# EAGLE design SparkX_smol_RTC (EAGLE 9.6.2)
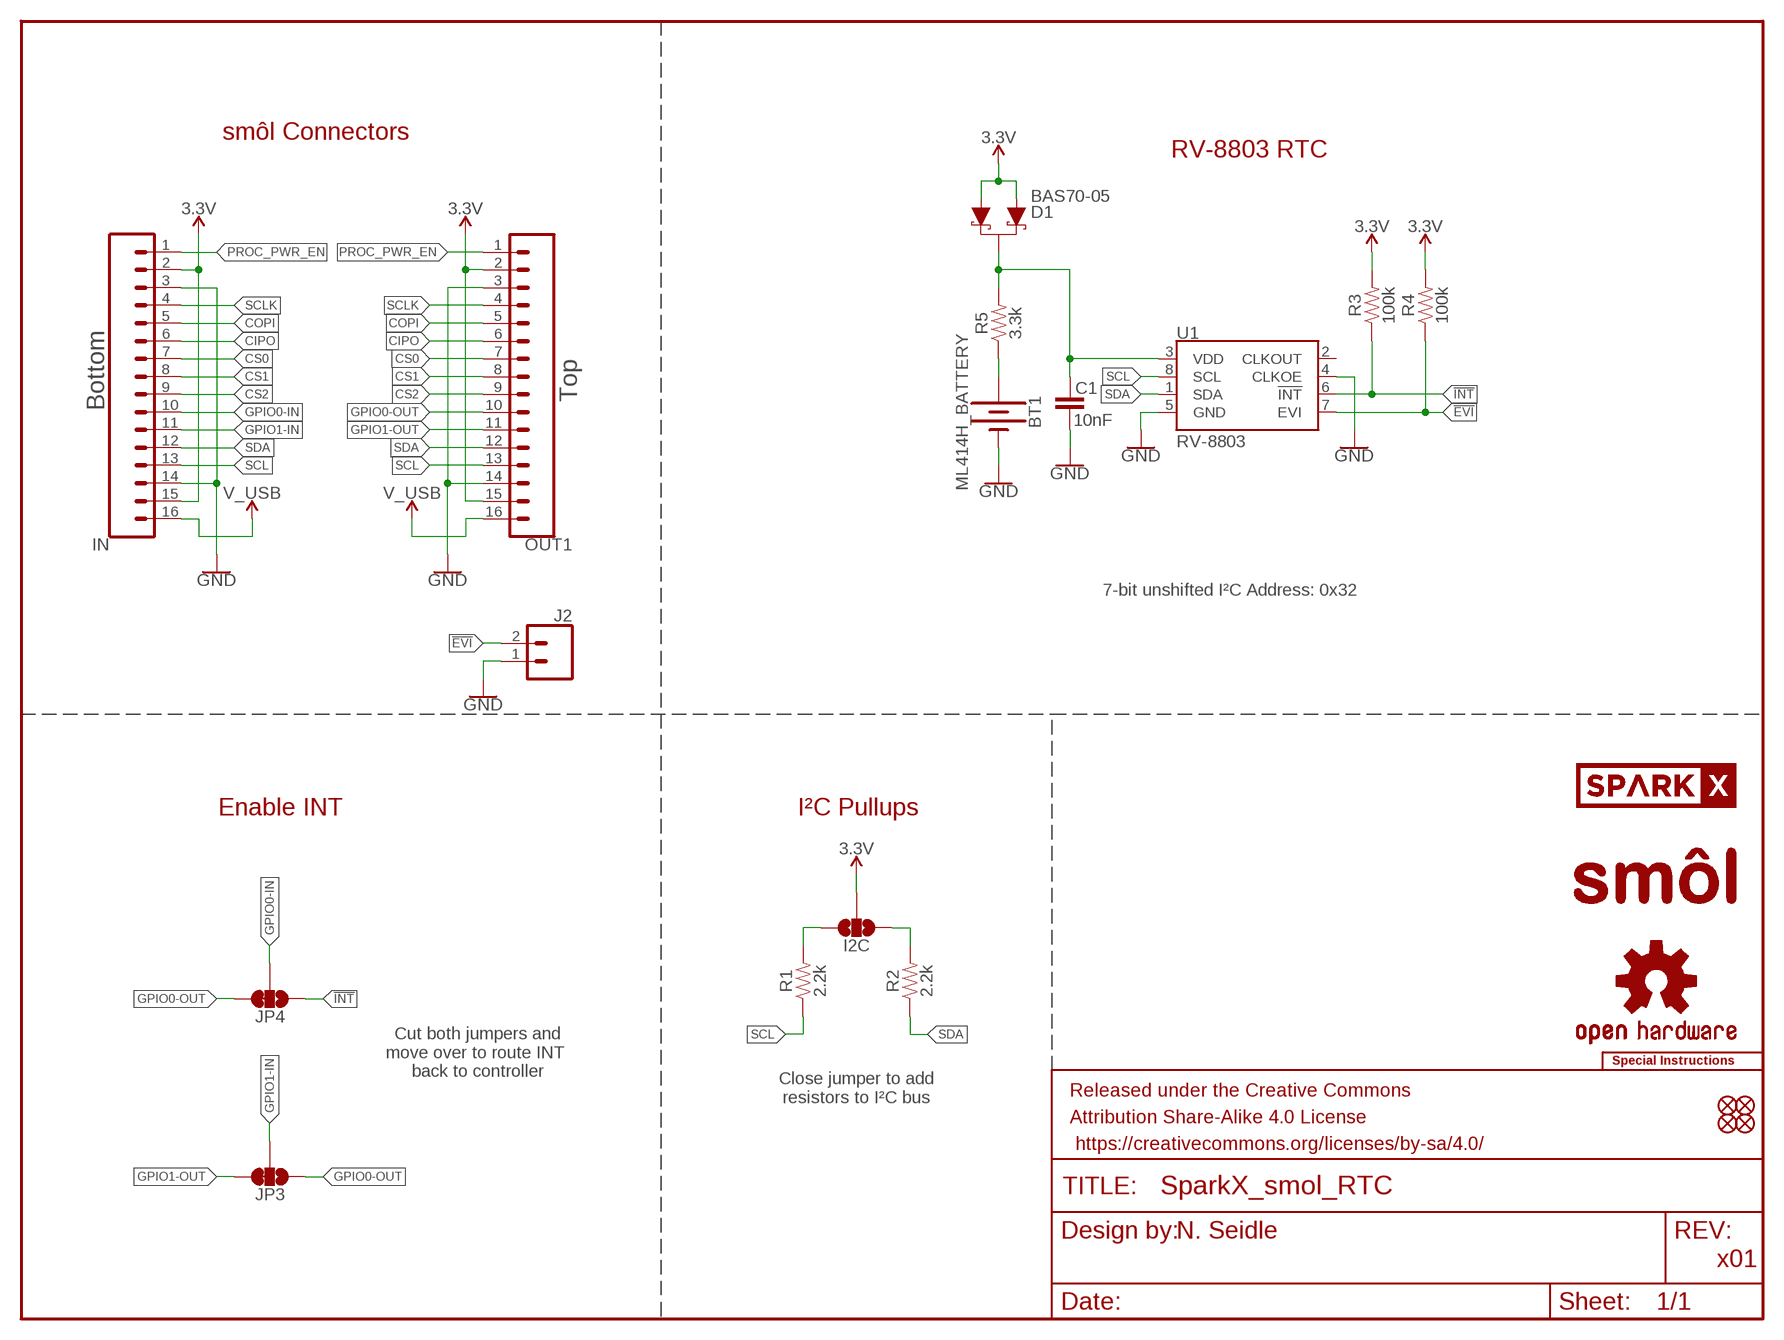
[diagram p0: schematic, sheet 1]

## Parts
BT1  ML414H_BATTERY  ML414H_IV01E_BATTERY  [ML414H_IV01E]
C1  10nF  10NF-0603-50V-10%  [0603]
D1  BAS70-05  DIODE-SCHOTTKY-DUAL  [SOT23-3@1]
FD1  FIDUCIALUFIDUCIAL  [FIDUCIAL-MICRO]
FD2  FIDUCIALUFIDUCIAL  [FIDUCIAL-MICRO]
FD3  FIDUCIALUFIDUCIAL  [FIDUCIAL-MICRO]
FD4  FIDUCIALUFIDUCIAL  [FIDUCIAL-MICRO]
FRAME2  FRAME-LETTER  [CREATIVE_COMMONS]
I2C  JUMPER-SMT_3_NO_SILK  [SMT-JUMPER_3_NO_SILK]
IN  CONN_16FPC_16_0.5MM  [FPC_16_0.5MM]
J2  CONN_021X02_NO_SILK  [1X02_NO_SILK]
JP3  JUMPER-SMT_3_1-NC_TRACE_SILK  [SMT-JUMPER_3_1-NC_TRACE_SILK]
JP4  JUMPER-SMT_3_1-NC_TRACE_SILK  [SMT-JUMPER_3_1-NC_TRACE_SILK]
LOGO1  SPECIAL_INSTRUCTIONS-ORDERING  [ORDERING_INSTRUCTIONS]
LOGO2  OSHW-LOGOMINI  [OSHW-LOGO-MINI]
OUT1  CONN_16FPC_16_0.5MM  [FPC_16_0.5MM]
R1  2.2k  2.2KOHM-0603-1/10W-1%  [0603@1]
R2  2.2k  2.2KOHM-0603-1/10W-1%  [0603@1]
R3  100k  100KOHM-0603-1/10W-1%  [0603@2]
R4  100k  100KOHM-0603-1/10W-1%  [0603@2]
R5  3.3k  3.3KOHM-0603-1/10W-1%  [0603]
U1  RV-8803  [RV-3028]
U$1  SPARKX-LOGO3  [SPARKX-SMALL]
U$39  SMOL_LOGOSMALL  [SMOL_SMALL]

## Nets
3.3V [power]: D1.1(A) D1.2(A1) I2C.2 IN.2 IN.15 OUT1.2 OUT1.15 R3.2 R4.2
!EVI: J2.2 R4.1 U1.7(EVI)
!INT: JP4.1 R3.1 U1.6(!INT)
CIPO: IN.6 OUT1.6
COPI: IN.5 OUT1.5
CS0: IN.7 OUT1.7
CS1: IN.8 OUT1.8
CS2: IN.9 OUT1.9
GND [power]: BT1.- C1.1 IN.3 IN.14 J2.1 OUT1.3 OUT1.14 U1.4(CLKOE) U1.5(GND)
GPIO0-IN: IN.10 JP4.2
GPIO0-OUT: JP3.1 JP4.3 OUT1.10
GPIO1-IN: IN.11 JP3.2
GPIO1-OUT: JP3.3 OUT1.11
N$1: I2C.3 R1.2
N$2: I2C.1 R2.2
N$4: BT1.+ R5.1
PROC_PWR_EN: IN.1 OUT1.1
SCL: IN.13 OUT1.13 R1.1 U1.8(SCL)
SCLK: IN.4 OUT1.4
SDA: IN.12 OUT1.12 R2.1 U1.1(SDA)
V_BACKUP: C1.2 D1.3(C) R5.2 U1.3(VDD)
V_USB [power]: IN.16 OUT1.16
Unconnected: U1.2(CLKOUT)

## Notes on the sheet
- smôl Connectors
- RV-8803 RTC
- Top
- Bottom
- 7-bit unshifted I²C Address: 0x32
- Enable INT | I²C Pullups
- Cut both jumpers and
  move over to route INT 
  back to controller
- Close jumper to add
  resistors to I²C bus
- N. Seidle
- x01

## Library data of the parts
BT1 = SparkFun-Batteries:ML414H_IV01E_BATTERY: SEIKO ML414H-IV01E Reflowable Lithium Battery; PROD_ID: BATT-14267
C1 = SparkFun-Capacitors:10NF: 0.01uF/10nF/10,000pF ceramic capacitors; PROD_ID: CAP-00867
D1 = SparkFun-DiscreteSemi:DIODE-SCHOTTKY-DUAL: Diodes Incorporated - BAS70-05 Dual Schottky Diode Two Schottky Diodes in a single SOT-23 package. Low reverse current (100 nA) Vf: Datasheet referenced for footprint; PROD_ID: DIO-14829
FD1-FD4 = SparkFun-Aesthetics:FIDUCIAL: Fiducial Alignment Points
FRAME2 = SparkFun-Aesthetics:FRAME-LETTER: Schematic Frame - Letter
I2C = SparkFun-Jumpers:JUMPER-SMT_3_NO: Normally open jumper This jumper has three pads in close proximity to each other. Apply solder to close the connection(s).
IN OUT1 = SparkFun-Connectors:CONN_16: Multi connection point. Often used as Generic Header-pin footprint for 0.1 inch spaced/style header connections On any of the 0.1 inch spaced packages, you can populate with these: Break Away Headers - Straight (PRT-00116) Break Away Male Headers - Right Angle (PRT-00553) Female Headers (PRT-00115)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; PROD_ID: CONN-16066
J2 = SparkFun-Connectors:CONN_02: Multi connection point. Often used as Generic Header-pin footprint for 0.1 inch spaced/style header connections
JP3 JP4 = SparkFun-Jumpers:JUMPER-SMT_3_1-NC_TRACE: Normally closed trace jumper (1 of 2 connections) This jumper has a trace between two pads so it's normally closed (NC). The other connection is normally open (NO). Use a razor knife to open the connection. For best results follow the IPC guidelines for cutting traces: Cutout at least 0.063 mm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
LOGO1 = SparkFun-Aesthetics:SPECIAL_INSTRUCTIONS: Special Ordering/Production Instructions Alert
LOGO2 = SparkFun-Aesthetics:OSHW-LOGO: Open-Source Hardware (OSHW) Logo
R1 R2 = SparkFun-Resistors:2.2KOHM: 2.2kΩ resistor; PROD_ID: RES-08272
R3 R4 = SparkFun-Resistors:100KOHM: 100kΩ resistor; PROD_ID: RES-07828
R5 = SparkFun-Resistors:3.3KOHM: 3.3kΩ resistor; PROD_ID: RES-07851
U1 = SparkFun-Clocks:RV-8803: Micro Crystal RV-8803 - Temperature compensated RTC Ultra accurate plus/minus 3PPM I2C RTC. Temperature compensated crystal for low drift; PROD_ID: IC-14828
U$1 = SparkX:SPARKX-LOGO
U$39 = SparkX:SMOL_LOGO

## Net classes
1 power: width 0.178 mm
2 3.3V: width 0.305 mm
3 VDDA: width 0.254 mm

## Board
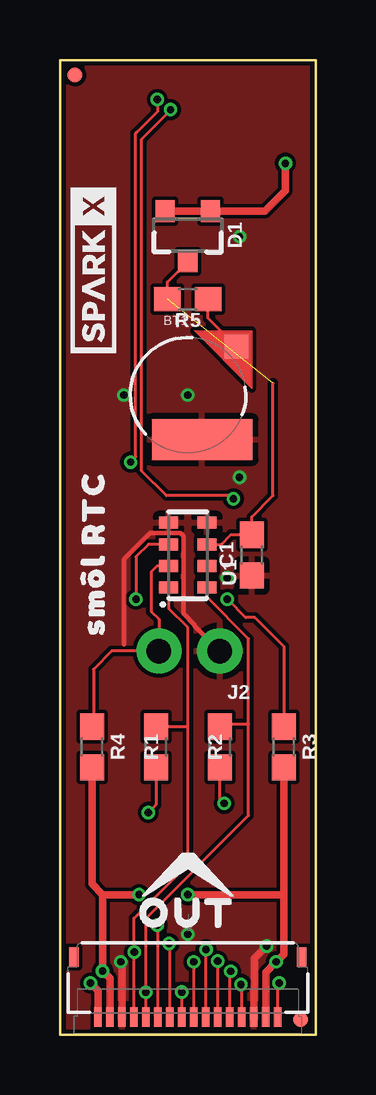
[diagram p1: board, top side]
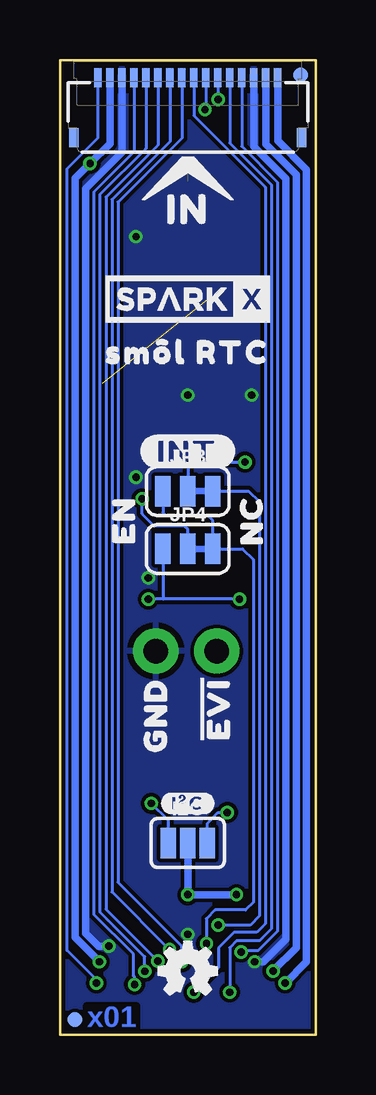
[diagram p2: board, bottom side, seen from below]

Size 10.67 x 40.64 mm. Coordinates in mm from the lower left corner, seen from the top.
Outline: 0,40.64 0,0 10.67,0 10.67,40.64 0,40.64
Copper layers (1*16): Top/Horz 0.035mm / dielectric 1.5mm / Bottom/Vert 0.035mm
Design rules "SparkFun-2-Layer-Minimum-JLCPCB": minimum track width 5mil, minimum drill 0.3mm, track to track 5mil, track to pad 5mil, pad to pad 5mil, via to via 5mil, smd to smd 5mil, copper to edge 7mil, drill to drill 7mil, minimum pad ring 5mil, minimum via ring 5mil, stop-mask expansion 2.5mil, vias tented up to drill 25mil, thermal gap 10mil

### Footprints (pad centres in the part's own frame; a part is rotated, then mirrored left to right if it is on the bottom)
ML414H_IV01E = smd 1 x 1: + 2.022,2.032 | smd 4.2 x 1.7: - 0.6,-1.85
0603 = smd 1.1 x 1: 1 -0.85,0; 2 0.85,0
SOT23-3@1 = smd 0.8 x 0.9: 1 -0.95,-1; 2 0.95,-1; 3 0,1.1
FIDUCIAL-MICRO = smd 0.635 x 0.635: 1 0,0
SMT-JUMPER_3_NO_SILK = smd 0.635 x 1.27: 1 -0.813,0; 2 0,0; 3 0.813,0
FPC_16_0.5MM = smd 0.3 x 0.8: 1 -3.75,1.35; 2 -3.25,1.35; 3 -2.75,1.35; 4 -2.25,1.35; 5 -1.75,1.35; 6 -1.25,1.35; 7 -0.75,1.35; 8 -0.25,1.35; 9 0.25,1.35; 10 0.75,1.35; 11 1.25,1.35; 12 1.75,1.35; 13 2.25,1.35; 14 2.75,1.35; 15 3.25,1.35; 16 3.75,1.35 | smd 0.4 x 0.8: MP1 -4.75,-1.15; MP2 4.75,-1.15
1X02_NO_SILK = drill 1.016 pad 1.88: 1 0,0; 2 2.54,0
SMT-JUMPER_3_1-NC_TRACE_SILK = smd 0.66 x 1.27: 1 -1.041,0; 2 0,0; 3 1.041,0
0603@1 = smd 1.1 x 1: 1 -0.85,0; 2 0.85,0
0603@2 = smd 1.1 x 1: 1 -0.85,0; 2 0.85,0
RV-3028 = smd 0.5 x 0.8: 1 -1.35,-0.8; 2 -0.45,-0.8; 3 0.45,-0.8; 4 1.35,-0.8; 5 1.35,0.8; 6 0.45,0.8; 7 -0.45,0.8; 8 -1.35,0.8

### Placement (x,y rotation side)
BT1  5.33,26.67 0 top
C1  8,20 90 top
D1  5.33,33.34 180 top
FD1  0.64,40.01 0 top
FD2  0.64,40.01 0 bottom
FD3  10.03,0.64 0 top
FD4  10.03,0.64 0 bottom
FRAME2  not placed on the board
I2C  5.33,8 0 bottom
IN  5.33,38.54 0 bottom
J2  6.67,16 180 top
JP3  5.33,22.67 0 bottom
JP4  5.33,20.26 0 bottom
LOGO1  not placed on the board
LOGO2  5.33,2.67 0 bottom
OUT1  5.33,2.1 180 top
R1  4,12 270 top
R2  6.67,12 270 top
R3  9.33,12 270 top
R4  1.33,12 270 top
R5  5.33,30.67 180 top
U1  5.33,20 90 top
U$1  1.4,31.88 90 top
U$2  [#EVI#0]  4.19,13.59 90 bottom
U$3  [GND0]  6.67,13.34 90 bottom
U$4  [SM�L_RTC0]  1.4,20.08 90 top
U$5  [SM�L_RTC0]  5.35,28.45 0 bottom
U$12  [IN0]  5.33,34.42 0 bottom
U$14  [EN1]  8,21.46 90 bottom
U$15  SMOL_LOGOSMALL  [SMOL_SMALL]  5.33,35.94 0 bottom
U$16  [#INT#0]  5.33,24.32 0 bottom
U$17  [NC2]  2.67,21.46 90 bottom
U$19  [#I�C#0]  5.33,9.65 0 bottom
U$20  SPARKX-LOGO3  [SPARKX-SMALL]  5.33,30.67 0 bottom
U$37  [OUT0]  5.33,5.08 0 top
U$39  5.33,6.92 0 top

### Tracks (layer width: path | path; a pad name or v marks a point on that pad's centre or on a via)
3.3V  (via drill 0.3)
  Top/Horz 0.305: OUT1.15 2.08,2.36 v1.78,2.67 1.78,4.06 1.78,4.32 1.78,5.84 | OUT1.2 8.58,2.62 v9.02,3.05 9.34,3.37 9.34,5.84 | R3.2 9.34,5.84 | v5.33,5.84 9.34,5.84 | D1.2 D1.1 8.56,34.34 9.41,35.19 v9.41,36.33 | R4.2 1.33,6.29 1.78,5.84 | 1.78,5.84 v3.3,5.84
  Bottom/Vert 0.305: v1.78,2.67 0.81,3.63 0.81,35.87 2.08,37.14 IN.15 | IN.2 8.58,37.16 v9.41,36.33 10.03,35.71 10.03,4.06 v9.02,3.05 | v3.3,5.84 v5.33,5.84 I2C.2
!EVI
  Top/Horz 0.127: R4.1 1.4,12.91 1.4,15.24 2.16,16 J2.2 4.13,17.34 3.81,17.65 3.81,19.3 4.06,19.55 U1.7
!INT  (via drill 0.3)
  Top/Horz 0.127: U1.6 3.69,20.45 3.17,19.94 v3.17,18.16 | R3.1 9.34,16.19 8.13,17.4 7.75,17.4 v6.99,18.16
  Bottom/Vert 0.127: v3.17,18.16 6.35,18.16 | 6.35,18.16 v6.99,18.16 | JP4.1 6.38,18.19 6.35,18.16
CIPO  (via drill 0.3)
  Top/Horz 0.127: v6.58,3.07 OUT1.6
  Bottom/Vert 0.127: v6.58,3.07 8.75,5.24 8.75,34.92 6.58,37.09 IN.6
COPI  (via drill 0.3)
  Top/Horz 0.127: OUT1.5 7.08,2.6 v7.13,2.65
  Bottom/Vert 0.127: v7.13,2.65 7.13,3.26 9,5.13 9,35.03 7.08,36.95 IN.5
CS0  (via drill 0.3)
  Top/Horz 0.127: OUT1.7 6.08,3.54 v6.1,3.56
  Bottom/Vert 0.127: v6.1,3.56 8.5,5.96 8.5,34.82 6.08,37.23 IN.7
CS1  (via drill 0.3)
  Top/Horz 0.127: OUT1.8 v5.58,3.04 v5.59,3.05
  Bottom/Vert 0.127: v5.59,3.05 5.59,3.71 8.24,6.37 8.24,34.71 5.58,37.37 IN.8
CS2  (via drill 0.3)
  Top/Horz 0.127: OUT1.9 v5.08,1.77 v5.08,1.78
  Bottom/Vert 0.127: IN.9 5.08,38.32 2.1,35.33 2.1,4.64 2.45,4.28 3.4,4.28 4.05,3.62 4.05,2.81 v5.08,1.78
GND  (via drill 0.3)
  Top/Horz 0.178: J2.1 5.61,17.06 5.61,17.1 5.15,17.56 5.15,20.79 5.02,20.92 3.76,20.92 2.68,19.84 2.68,16.29 2.67,16.28
  Top/Horz 0.305: OUT1.14 2.58,3 v2.54,3.05 | OUT1.3 8.08,1.84 8.11,1.87 8.11,3.19 v8.62,3.7
  Bottom/Vert 0.305: v2.54,3.05 2.19,3.05 1.25,3.99 1.25,35.69 2.58,37.02 IN.14 | v8.62,3.7 9.05,3.7 9.6,4.24 9.6,35.28 8.08,36.79 IN.3
  other vias: 5.33,4.19 5.33,26.67 6.99,19.05 7.49,23.24 7.49,33.27 2.67,26.67
  pour Top/Horz (isolate 0.152, rank 3): 0,40.64 10.67,40.64 10.67,0 0,0
  pour Bottom/Vert (isolate 0.152, rank 2): 0,40.64 10.67,40.64 10.67,0 0,0
GPIO0-IN  (via drill 0.3)
  Top/Horz 0.127: v4.61,38.57 4.61,38.55 3.42,37.35 3.42,23.51 4.45,22.48 7.11,22.48 v7.24,22.35
  Bottom/Vert 0.127: JP4.2 5.33,21.08 5.46,21.21 6.73,21.21 7.24,21.72 v7.24,22.35 | IN.10 4.58,38.6 v4.61,38.57
GPIO0-OUT  (via drill 0.3)
  Top/Horz 0.127: OUT1.10 4.58,3.78 v4.55,3.81
  Bottom/Vert 0.127: v4.55,3.81 4.55,4.84 4.19,5.21 2.92,5.21 2.6,5.52 2.6,19.81 3.05,20.26 JP4.3 4.29,21.44 4.51,21.65 6.25,21.65 6.38,21.78 JP3.1
GPIO1-IN  (via drill 0.3)
  Top/Horz 0.127: v4.06,38.99 4.06,38.48 3.24,37.66 3.16,37.58 3.16,24.09 v2.95,23.88
  Bottom/Vert 0.127: IN.11 4.08,39.01 v4.06,38.99 | JP3.2 5.33,23.65 5.11,23.88 v2.95,23.88 | v2.95,23.88
GPIO1-OUT  (via drill 0.3)
  Top/Horz 0.127: OUT1.11 4.08,4.55 v4.06,4.57
  Bottom/Vert 0.127: JP3.3 2.79,22.67 2.35,22.23 2.35,4.95 2.73,4.57 v4.06,4.57
N$1  (via drill 0.3)
  Top/Horz 0.127: v3.68,9.27 4,9.59 R1.2
  Bottom/Vert 0.127: v3.68,9.27 4.06,9.27 4.52,8.81 I2C.3
N$2  (via drill 0.3)
  Top/Horz 0.127: v6.86,9.65 6.67,9.65 R2.2
  Bottom/Vert 0.127: v6.86,9.65 6.15,8.94 I2C.1
N$4
  Top/Horz 0.127: BT1.+ 6.18,29.87 R5.1
PROC_PWR_EN  (via drill 0.3)
  Top/Horz 0.127: OUT1.1 9.08,2.1 v9.14,2.16
  Bottom/Vert 0.127: v9.14,2.16 9.14,2.29 10.38,3.52 10.38,36.11 9.08,37.4 IN.1
SCL  (via drill 0.3)
  Top/Horz 0.127: OUT1.13 3.08,3.43 | 3.08,3.43 3.08,4.86 5.33,7.11 5.33,12.83 | v3.11,3.45 3.08,3.43 | U1.8 4.53,17.78 5.33,16.98 5.33,12.83 | R1.1 5.31,12.85 5.33,12.83
  Bottom/Vert 0.127: IN.13 3.08,37.04 1.59,35.54 1.59,4.32 2.39,3.52 3.04,3.52 v3.11,3.45
SCLK  (via drill 0.3)
  Top/Horz 0.127: OUT1.4 7.58,2.07 v7.55,2.1
  Bottom/Vert 0.127: v7.55,2.1 7.55,2.41 7.6,2.46 7.6,3.37 9.26,5.03 9.26,35.13 7.58,36.81 IN.4
SDA  (via drill 0.3)
  Top/Horz 0.127: OUT1.12 v3.58,1.78 3.58,4.85 7.87,9.14 7.87,12.95 | 7.87,12.95 7.87,16.51 6.13,18.25 U1.1 | R2.1 6.77,12.95 7.87,12.95
  Bottom/Vert 0.127: IN.12 3.58,37.18 1.84,35.44 1.84,4.42 2.34,3.92 3.3,3.92 3.58,3.64 v3.58,1.78
V_BACKUP  (1 unrouted)
  Top/Horz 0.127: U1.3 6.74,20.45 7.14,20.85 C1.2 8,21.59 8.89,22.48 8.89,27.17 | R5.2 4.48,31.39 D1.3
V_USB  (via drill 0.3)
  Top/Horz 0.305: v1.27,2.16 1.58,1.84 OUT1.16
  Bottom/Vert 0.305: IN.16 1.58,37.27 0.38,36.07 0.38,3.05 v1.27,2.16

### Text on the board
Bottom/Vert: x01
Measures: Dimensions in Inches
tDocu: 2-Layer Board / 0.8mm Thickness / 1oz Copper | N. Seidle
